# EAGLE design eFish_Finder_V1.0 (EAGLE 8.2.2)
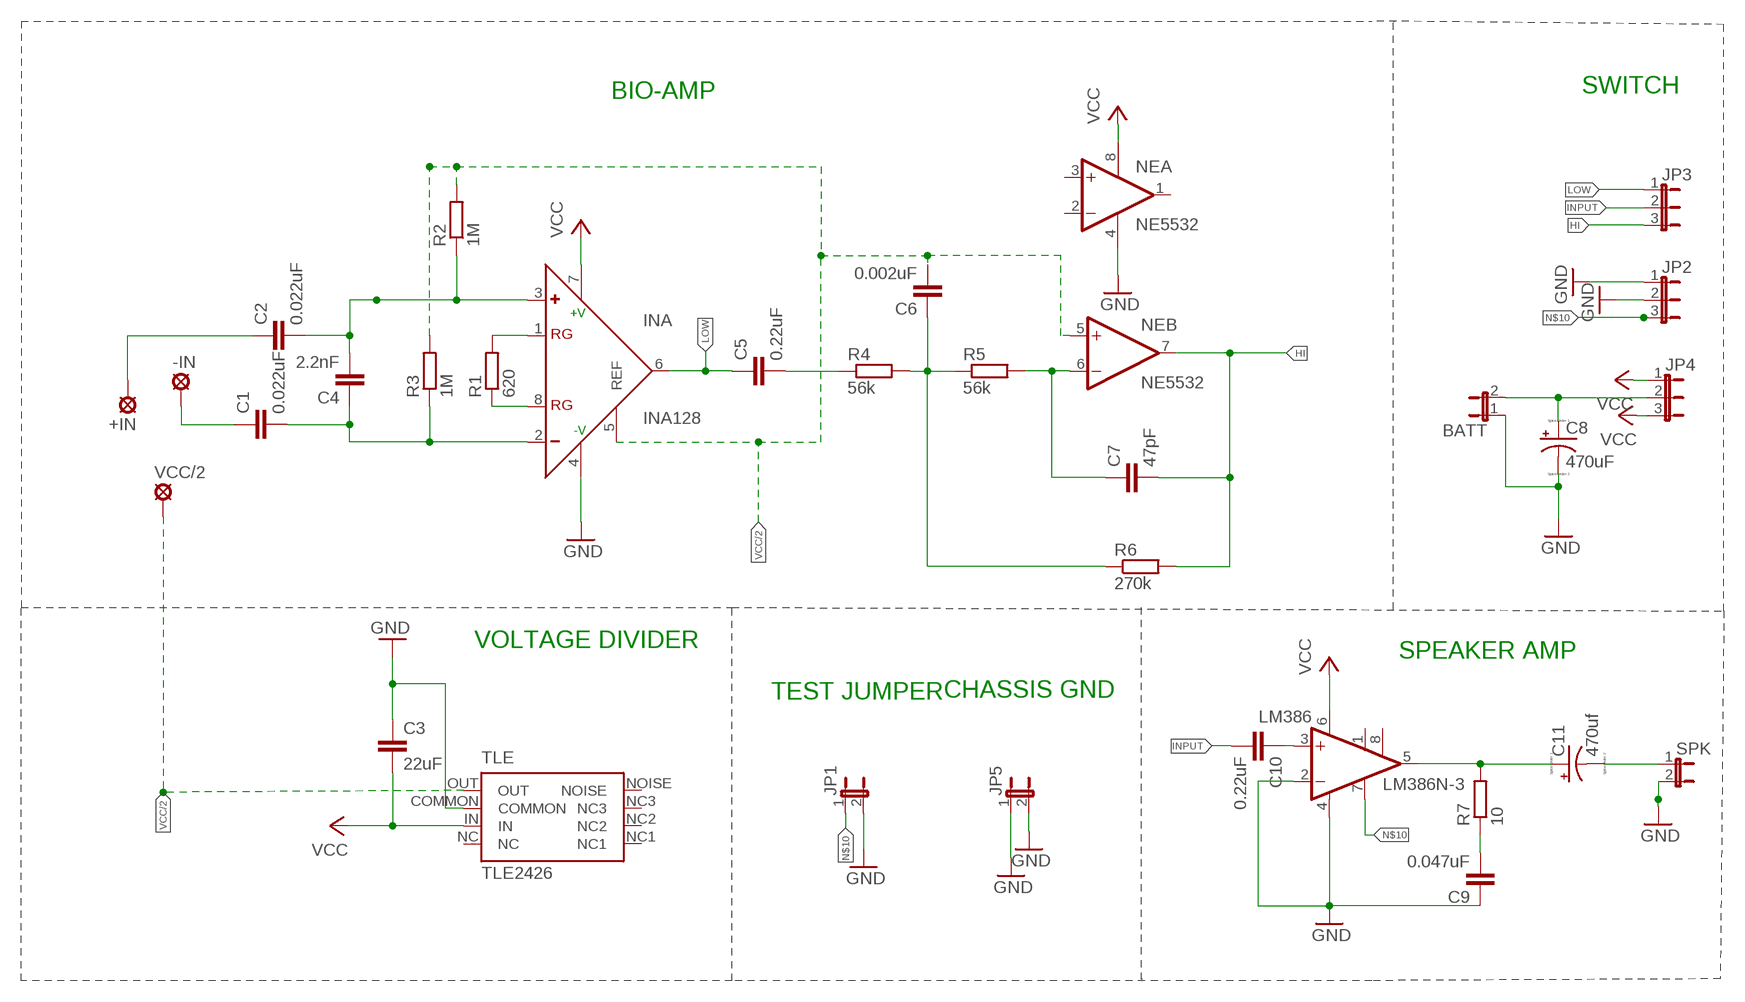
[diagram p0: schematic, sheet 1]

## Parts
+IN  LSP11  [LSP11]
-IN  LSP11  [LSP11]
BATT  JP1E  [JP1]
C1  0.022uF  C-EU025-025X050  [C025-025X050]
C2  0.022uF  C-EU025-025X050  [C025-025X050]
C3  22uF  C-EU025-025X050  [C025-025X050]
C4  2.2nF  C-EU025-025X050  [C025-025X050]
C5  0.22uF  C-EU025-025X050  [C025-025X050]
C6  0.002uF  C-EU025-025X050  [C025-025X050]
C7  47pF  C-EU025-025X050  [C025-025X050]
C8  470uF  CPOL-USE5-10.5  [E5-10,5]
C9  0.047uF  C-EU025-025X050  [C025-025X050]
C10  0.22uF  C-EU025-025X050  [C025-025X050]
C11  470uf  CPOL-USE5-10.5  [E5-10,5]
INA  INA128  AD623N  [DIL08]
JP1  JP1E  [JP1]
JP2  JP2E  [JP2]
JP3  JP2E  [JP2]
JP4  JP2E  [JP2]
JP5  JP1E  [JP1]
LM386  LM386N-3  [DIL08]
NE  NE5532  TLC272P  [DIL08]
R1  620  R-EU_0207/2V  [0207/2V]
R2  1M  R-EU_0207/2V  [0207/2V]
R3  1M  R-EU_0207/2V  [0207/2V]
R4  56k  R-EU_0207/2V  [0207/2V]
R5  56k  R-EU_0207/2V  [0207/2V]
R6  270k  R-EU_0207/2V  [0207/2V]
R7  10  R-EU_0207/2V  [0207/2V]
SPK  JP1E  [JP1]
TLE  TLE2426  [DIL08]
VCC/2  LSP11  [LSP11]

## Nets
GND: BATT.1 C3.1 C8.- C9.1 INA.4(-V) JP1.2 JP2.1 JP2.2 JP5.1 JP5.2 LM386.2(-IN) LM386.4(GND) NE.4(P:V-) SPK.2 TLE.COMMON
HI: C7.2 JP3.3 NE.7(B:OUT) R6.2
INPUT: C10.2 JP3.2
LOW: C5.1 INA.6(OUT) JP3.1
N$1: C11.- SPK.1
N$2: +IN.MP C2.1
N$3: -IN.MP C1.1
N$4: C1.2 C4.1 INA.2(-) R3.1
N$5: INA.8(RG) R1.1
N$6: INA.1(RG) R1.2
N$7: C5.2 R4.1
N$8: C6.1 R4.2 R5.1 R6.1
N$9: C7.1 NE.6(B:-IN) R5.2
N$10: JP1.1 JP2.3 LM386.7(BYPASS)
N$12: C9.2 R7.1
N$13: C11.+ LM386.5(OUT) R7.2
N$14: C10.1 LM386.3(+IN)
N$17: C2.2 C4.2 INA.3(+) R2.1
N$19: BATT.2 C8.+ JP4.2
VCC: C3.2 INA.7(+V) JP4.1 JP4.3 LM386.6(VS) NE.8(P:V+) TLE.IN
VCC/2: C6.2 INA.5(REF) NE.5(B:+IN) R2.2 R3.2 TLE.OUT VCC/2.MP
Unconnected: LM386.1(GAIN) LM386.8(GAIN) NE.1(A:OUT) NE.2(A:-IN) NE.3(A:+IN) TLE.NC1 TLE.NC2 TLE.NC3 TLE.NOISE

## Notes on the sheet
- BIO-AMP | SWITCH
- VOLTAGE DIVIDER
- SPEAKER AMP
- TEST JUMPER | CHASSIS GND

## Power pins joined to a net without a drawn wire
NC: TLE.NC

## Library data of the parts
+IN -IN VCC/2 = solpad:LSP11: SOLDER PAD
BATT JP1 JP5 SPK = jumper:JP1E: JUMPER
C1-C7 C9 C10 = rcl:C-EU: CAPACITOR, European symbol
C8 C11 = resistor:CPOL-US: POLARIZED CAPACITOR, American symbol
INA = analog-devices:AD623: Single-Supply, Rail-to-Rail, Low Cost Instrumentation Amplifier Source: http://www.analog.com/static/imported-files/data_sheets/AD623.pdf; MF: ALTERA CORPORATION; MPN: AD623ANZ; OC_FARNELL: 9603700; OC_NEWARK: 59K4402
JP2-JP4 = jumper:JP2E: JUMPER
LM386 = linear:LM386?-*: Low Voltage Audio Power Amplifier Source: http://cache.national.com/ds/LM/LM386.pdf
NE = linear:TLC272: OP AMP
R1-R7 = rcl:R-EU_: RESISTOR, European symbol
TLE = TLE2426:TLE2426

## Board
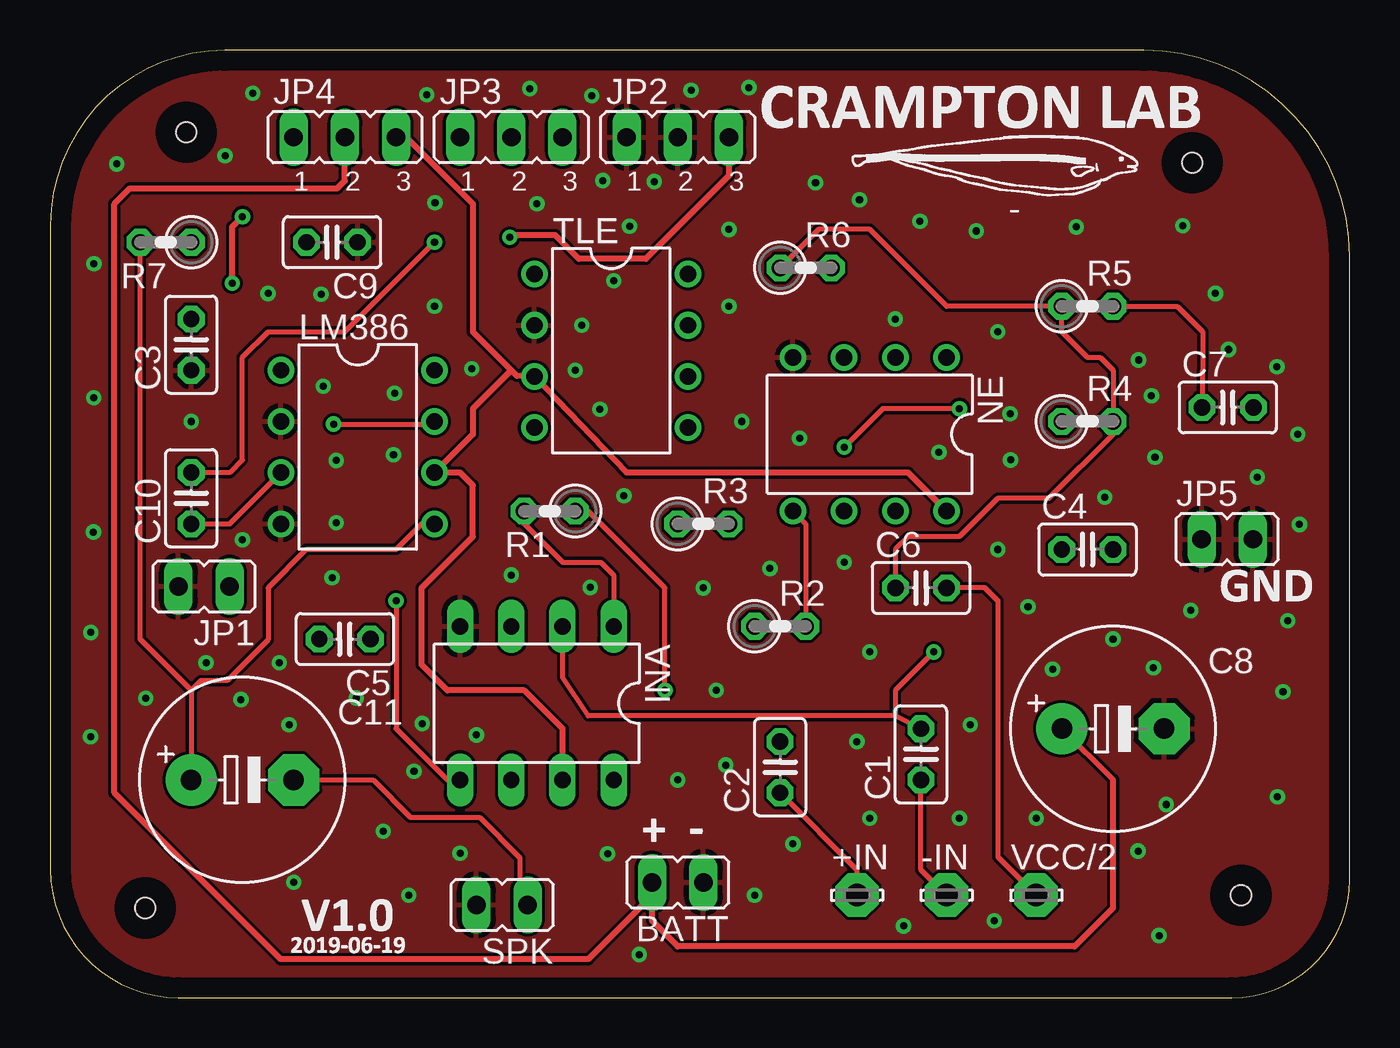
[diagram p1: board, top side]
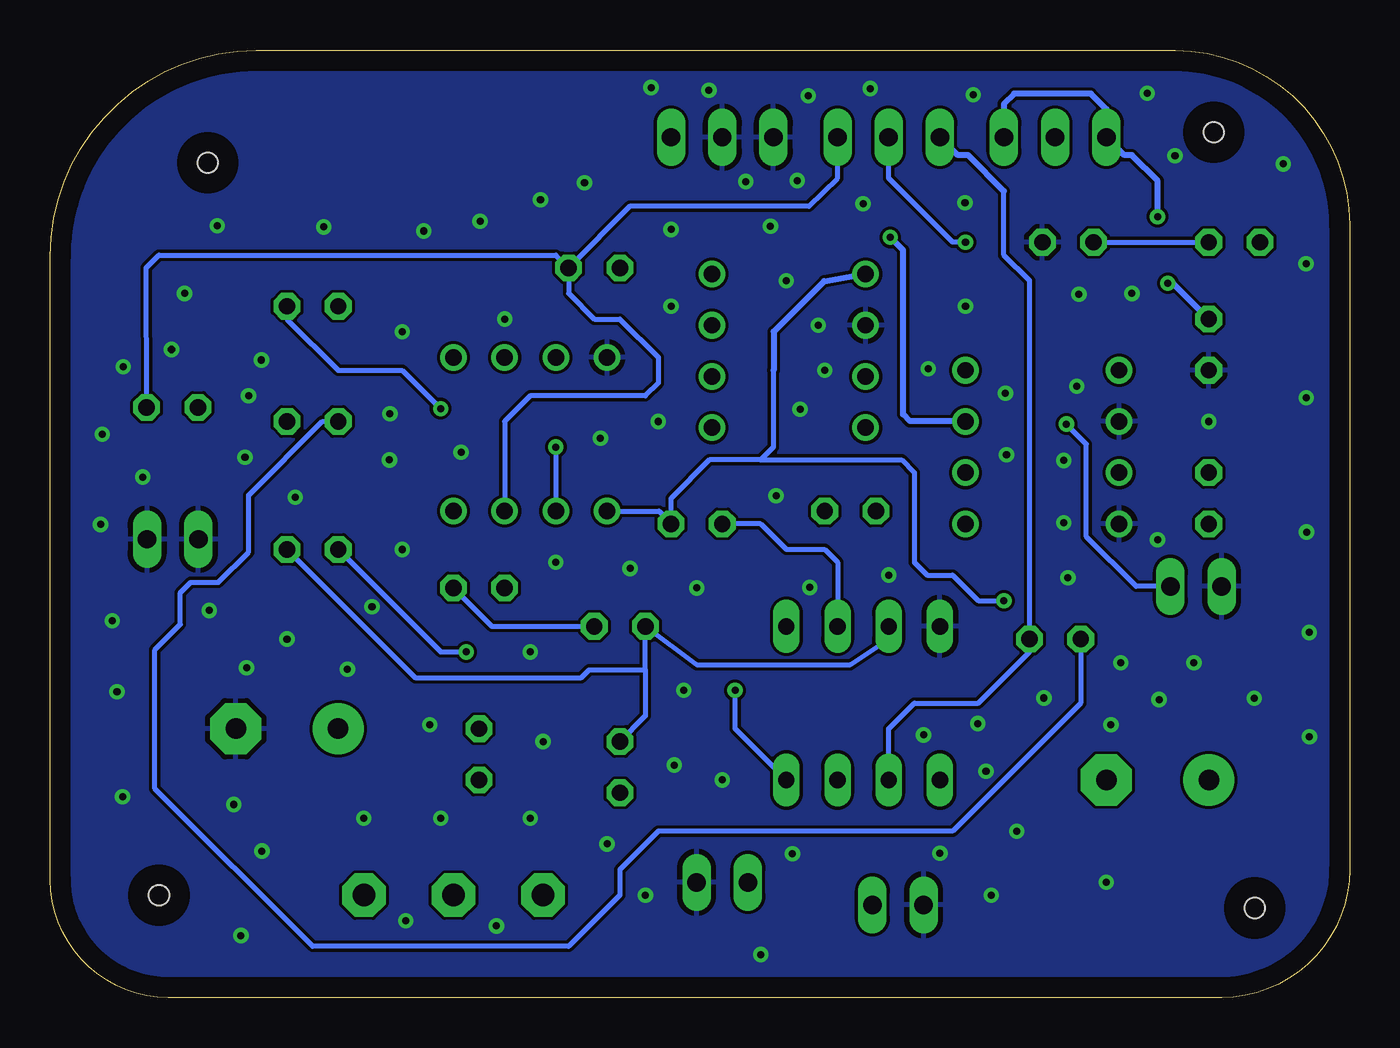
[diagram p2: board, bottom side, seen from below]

Size 64.44 x 46.98 mm. Coordinates in mm from the lower left corner, seen from the top.
Outline: 0,38.32 0,6.35 arc90 6.35,0 58.59,0 arc90 64.44,5.85 64.44,36.77 arc90 54.23,46.98 8.65,46.98 arc90 0,38.32
Copper layers (1*16): Top 0.035mm / dielectric 1.5mm / Bottom 0.035mm
Design rules "default": minimum track width 6mil, minimum drill 0.35mm, track to track 6mil, track to pad 6mil, pad to pad 6mil, via to via 6mil, smd to smd 6mil, copper to edge 40mil, drill to drill 6mil, minimum pad ring 10mil, minimum via ring 8mil, stop-mask expansion 4mil, vias tented up to drill 0mil, thermal gap 10mil
Holes 1 mm at 4.7,4.45 6.73,42.93 56.64,41.4 59.05,5.08

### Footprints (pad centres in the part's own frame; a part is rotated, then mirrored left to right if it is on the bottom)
LSP11 = drill 1.118 pad 2.159 octagon: MP 0,0
JP1 = drill 0.914 long: 1 0,-1.27; 2 0,1.27
C025-025X050 = drill 0.813 octagon: 1 -1.27,0; 2 1.27,0
E5-10,5 = drill 1.016 pad 2.54: + -2.54,0 | drill 1.016 pad 2.54 octagon: - 2.54,0
DIL08 = drill 0.813 long: 1 -3.81,-3.81; 2 -1.27,-3.81; 3 1.27,-3.81; 4 3.81,-3.81; 5 3.81,3.81; 6 1.27,3.81; 7 -1.27,3.81; 8 -3.81,3.81
JP2 = drill 0.914 long: 1 -2.54,0; 2 0,0; 3 2.54,0
DIL08' = drill 0.813 pad 1.27: 1 -3.81,-3.81; 2 -1.27,-3.81; 3 1.27,-3.81; 4 3.81,-3.81; 5 3.81,3.81; 6 1.27,3.81; 7 -1.27,3.81; 8 -3.81,3.81
0207/2V = drill 0.813 octagon: 1 -1.27,0; 2 1.27,0
DIL08'' = drill 0.813 pad 1.27: COMMON -1.27,-3.81; IN 1.27,-3.81; NC 3.81,-3.81; NC1 3.81,3.81; NC2 1.27,3.81; NC3 -1.27,3.81; NOISE -3.81,3.81; OUT -3.81,-3.81

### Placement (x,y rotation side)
+IN  40.01,5.08 0 top
-IN  44.45,5.08 0 top
BATT  31.12,5.71 90 top
C1  43.18,12.06 90 top
C2  36.2,11.43 90 top
C3  6.99,32.38 90 top
C4  51.44,22.23 0 top
C5  14.61,17.78 180 top
C6  43.18,20.32 0 top
C7  58.39,29.27 0 top
C8  52.7,13.33 0 top
C9  13.97,37.47 180 top
C10  6.99,24.77 90 top
C11  9.52,10.79 0 top
INA  24.13,14.6 180 top
JP1  7.62,20.4 90 top
JP2  31.12,42.67 0 top
JP3  22.86,42.67 0 top
JP4  14.61,42.67 0 top
JP5  58.37,22.73 270 top
LM386  LM386N-3  [DIL08']  15.24,27.3 270 top
NE  NE5532  [DIL08']  40.64,27.94 180 top
R1  24.77,24.13 180 top
R2  36.2,18.41 0 top
R3  32.38,23.5 0 top
R4  51.44,28.58 0 top
R5  51.44,34.29 0 top
R6  37.47,36.2 0 top
R7  5.72,37.47 180 top
SPK  22.4,4.6 90 top
TLE  TLE2426  [DIL08'']  27.81,32.08 270 top
VCC/2  48.9,5.08 0 top

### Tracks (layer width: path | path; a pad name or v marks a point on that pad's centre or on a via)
GND  (via drill 0.35)
  other vias: 7.72,16.61 22.86,20.95 16.51,8.26 31.12,10.79 47.62,26.67 33.66,34.29 19.05,34.29 13.54,30.33 10.79,34.93 24.13,39.37 37.95,40.41 33.66,38.1 6.99,28.58 32.38,20.32 52.7,17.78 46.99,22.23 39.37,21.59 34.29,28.58 41.91,33.66 45.92,38.02 34.93,5.08 45.09,8.89 48.9,8.89 40.64,8.89 36.83,7.62 17.78,5.08 12.07,5.71 26.04,31.12 27.94,35.56 46.99,33.02 57.79,34.93 54.61,29.84 33.02,15.24 40.64,17.15 40.01,12.7 40.13,39.57 13.97,20.83 28.45,24.89 17.02,26.92 61.37,18.69 56.57,19.2 43.13,38.51 50.88,38.23 56.16,38.28 60.83,31.29 61.87,27.94 61.14,15.16 60.86,9.96 54.99,3.07 46.81,3.81 42.32,3.56 29.21,2.13 33.5,11.53 20.32,7.16 27.64,7.14 21.13,13.03 26.77,20.35 37.16,27.74 44.07,27.05 47.6,28.96 53.98,31.62 54.71,16.36 49.71,16.28 14.17,26.64 14.17,23.55 9.45,14.78 18.67,44.78 26.85,44.73 34.65,45.14 31.78,45.01 23.77,45.09 10.03,44.86 8.66,41.76 19.08,39.42 52.3,24.82 35.69,21.29 20.9,31.19 17.07,29.97 55.35,9.58 18.03,11.23 18.44,13.59 15.16,14.86 11.84,13.54 45.62,13.54 48.49,19.38 61.95,23.47 54.79,26.8 58.43,32.14 53.95,7.26 9.52,22.71 11.35,16.61 28.73,38.25 27.25,29.18 59.86,25.82 2.16,36.4 2.15,29.76 2.13,23.09 2.01,18.11 4.72,14.85 1.99,12.94 3.29,41.35 26.35,33.35 27.39,40.53 29.95,40.47 13.42,34.89
  pour Top: -1.91,-0.63 -1.91,42.55 2.54,46.99 60.33,46.99 65.4,41.91 65.4,3.81 60.33,-1.27 -1.27,-1.27
  pour Bottom: -1.91,-0.63 -1.91,42.55 2.54,46.99 60.33,46.99 65.4,41.91 65.4,3.81 60.33,-1.27 -1.27,-1.27
HI
  Bottom 0.254: C7.2 59.69,36.19 59.05,36.83 39.37,36.83 R6.2 | R6.2 35.71,39.24 26.82,39.24 25.4,40.64 JP3.3 | R6.2 38.73,34.92 37.46,33.65 36.19,33.65 34.29,31.75 34.29,30.48 34.92,29.84 40.64,29.84 41.91,28.57 NE.7
INPUT  (via drill 0.35)
  Top 0.254: v19.05,37.46 14.6,33.02 10.79,33.02 9.52,31.75 9.52,26.67 8.89,26.03 C10.2
  Bottom 0.254: v19.05,37.46 19.68,37.46 22.86,40.64 JP3.2
LOW
  Bottom 0.254: 17.14,40 17.14,36.83 15.87,35.56 C5.1 15.87,17.14 18.41,14.6 21.59,14.6 22.86,13.33 INA.6
  Bottom 0.305: 17.14,40 18.92,41.78 19.43,41.78 JP3.1
N$1
  Top 0.254: C11.- 16,10.79 17.86,8.94 21.29,8.94 23.29,6.93 23.29,4.98 SPK.1
N$2
  Top 0.254: C2.1 40,6.35 +IN.MP
N$3
  Top 0.254: -IN.MP 43.18,6.35 C1.1
N$4  (via drill 0.35)
  Top 0.254: 41.91,13.97 C1.2 | INA.2 25.4,15.87 26.67,13.97 41.91,13.97 | v43.81,17.14 41.91,15.24 41.91,13.97
  Bottom 0.254: C4.1 45.08,17.14 v43.81,17.14 | R3.1 29.21,23.49 27.94,22.22 26.03,22.22 25.4,21.59 INA.2
N$5  (via drill 0.35)
  Top 0.254: v30.48,15.24 30.48,20.32 26.67,24.13 R1.1
  Bottom 0.254: INA.8 30.48,13.33 v30.48,15.24
N$6
  Top 0.254: R1.2 23.49,23.49 25.4,21.59 27.3,21.59 27.94,20.95 INA.1
N$7
  Bottom 0.254: C5.2 13.33,14.6 19.68,8.25 34.29,8.25 36.19,6.35 36.19,5.08 38.73,2.54 51.43,2.54 59.26,10.36 59.26,17.25 57.99,18.52 57.99,20.09 57.48,20.6 56.11,20.6 54.61,22.1 54.61,24.92 50.95,28.57 R4.1
N$8
  Top 0.254: C6.1 41.91,22.22 42.54,22.86 45.08,22.86 46.99,24.76 49.53,24.76 52.7,27.94 R4.2 52.7,31.11 52.07,31.75 51.43,31.75 50.16,33.02 R5.1 44.45,34.29 40.64,38.1 38.1,38.1 R6.1
N$9  (via drill 0.35)
  Top 0.254: R5.2 55.88,34.29 57.15,33.02 C7.1 | v45.08,29.21 41.27,29.21 v39.37,27.3
  Bottom 0.254: R5.2 52.7,33.65 50.16,31.11 46.99,31.11 v45.08,29.21 | v39.37,27.3 NE.6
N$10  (via drill 0.35)
  Top 0.254: v14.05,28.45 18.92,28.45 LM386.7
  Top 0.305: JP2.3 33.65,40.75 29.54,36.64 26.21,36.64 25.03,37.82 22.9,37.82 v22.78,37.71
  Bottom 0.254: JP1.1 10.59,20.4 13.06,22.86 13.06,27.46 v14.05,28.45
  Bottom 0.305: LM386.7 19.06,28.59 21.81,28.59 22.15,28.93 22.15,37.07 v22.78,37.71
N$12
  Bottom 0.254: C9.2 R7.1
N$13
  Top 0.254: R7.2 4.44,17.78 6.98,15.24 | LM386.5 18.41,23.49 17.14,22.22 12.7,22.22 10.79,20.32 10.79,17.75 8.76,15.72 7.47,15.72 6.98,15.24 | 6.98,15.24 C11.+
N$14
  Top 0.254: C10.1 8.89,23.49 LM386.3
N$17
  Bottom 0.254: C2.2 34.92,13.97 34.92,16.25 | 34.92,16.25 R2.1 32.38,16.51 24.76,16.51 22.86,17.78 INA.3 | C4.2 46.35,15.87 38.1,15.87 37.72,16.25 34.92,16.25
N$19
  Top 0.254: 52.7,10.79 C8.+
  Top 0.305: 52.7,10.79 52.7,4.44 50.8,2.54 31.11,2.54 29.84,3.81 BATT.2 29.84,5.08 26.67,1.9 11.43,1.9 3.17,10.16 3.17,39.37 3.94,40.13 14.22,40.13 14.6,40.51 JP4.2
VCC  (via drill 0.35)
  Top 0.305: 22.86,31.11 20.95,33.02 20.95,39.37 17.65,42.67 JP4.3 | 22.86,31.11 20.95,29.21 20.95,27.94 LM386.6 20.32,26.03 20.95,25.4 20.95,22.86 18.41,20.32 18.41,16.51 19.68,15.24 23.49,15.24 25.4,13.33 INA.7 | NE.8 42.54,26.03 28.57,26.03 TLE.IN 23.14,30.84 22.86,31.11 | v9.02,35.43 9.02,38.23 v9.52,38.73
  Bottom 0.305: v9.52,38.73 9.52,40.51 10.79,41.78 11.18,41.78 JP4.1 12.06,44.07 12.83,44.83 16.64,44.83 17.14,44.32 JP4.3 | v9.02,35.43 8.76,35.43 C3.2
VCC/2  (via drill 0.35)
  Top 0.254: C6.2 46.35,20.32 46.99,19.68 46.99,6.98 VCC/2.MP | NE.5 37.46,23.49 R2.2 | v17.14,19.68 17.14,13.33 19.68,10.79 INA.5
  Bottom 0.254: 28.57,31.11 28.57,27.3 29.21,26.67 | 29.21,26.67 31.75,26.67 33.65,24.76 33.65,23.54 | 33.65,23.54 R3.2 | C6.2 42.54,18.41 R2.2 | 29.21,26.67 22.22,26.67 21.59,26.03 21.59,21.59 20.95,20.95 19.68,20.95 18.41,19.68 v17.14,19.68 | NE.5 34.25,24.13 33.65,23.54
  Bottom 0.305: 28.57,31.11 28.56,31.13 28.56,33.03 26.06,35.53 TLE.OUT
